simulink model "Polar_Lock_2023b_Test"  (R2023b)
settings: Solver=FixedStepDiscrete  StartTime=0.0  StopTime=inf  FixedStep=0.01  RelTol=1e-3  EnableMultiTasking=on
libraries: arduinolib x7

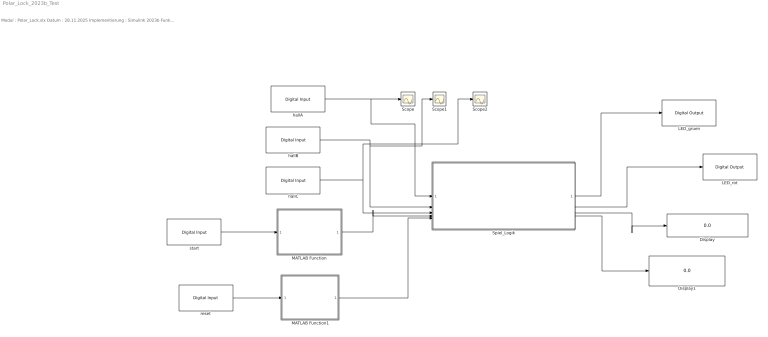
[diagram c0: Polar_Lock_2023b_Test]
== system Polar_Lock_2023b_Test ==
  note: Modul : Polar_Lock.slx Datum : 28.11.2025 Implementierung : Simulink 2023b Funktion: Autor : Yash Uppal und Barinder Singh Letzte Änderung : 28.12.2025
  Display : Display
  Display1 : Display
  LED_gruen : arduinolib/Digital Output  pinNumber=11  Direction=output  blockPlatform=arduino
  LED_rot : arduinolib/Digital Output  pinNumber=12  Direction=output  blockPlatform=arduino
  MATLAB Function : MATLAB Function  TreatAsAtomicUnit=on
  MATLAB Function1 : MATLAB Function  TreatAsAtomicUnit=on
  Scope : Scope
  Scope1 : Scope
  Scope2 : Scope
  Spiel_Logik : Subsystem
  hallA : arduinolib/Digital Input  pinNumber=3  mode=Default  Direction=input  SampleTime=0.1  blockPlatform=arduino
  hallB : arduinolib/Digital Input  pinNumber=4  mode=Default  Direction=input  SampleTime=0.1  blockPlatform=arduino
  hallC : arduinolib/Digital Input  pinNumber=6  mode=Default  Direction=input  SampleTime=0.1  blockPlatform=arduino
  reset : arduinolib/Digital Input  pinNumber=9  mode=Default  Direction=input  SampleTime=0.1  blockPlatform=arduino
  start : arduinolib/Digital Input  pinNumber=8  mode=Default  Direction=input  SampleTime=0.1  blockPlatform=arduino
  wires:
  hallA/1 -> Spiel_Logik/1(hallA), Scope/1
  hallB/1 -> Spiel_Logik/2(hallB), Scope1/1
  hallC/1 -> Spiel_Logik/3(hallC), Scope2/1
  Spiel_Logik/1(LED_gruen) -> LED_gruen/1
  Spiel_Logik/2(LED_rot) -> LED_rot/1
  Spiel_Logik/3(code) -> Display/1
  Spiel_Logik/4(status) -> Display1/1
  start/1 -> MATLAB Function/1(startRaw)
  MATLAB Function/1(startEvent) -> Spiel_Logik/4(startEvent)
  reset/1 -> MATLAB Function1/1(resetRaw)
  MATLAB Function1/1(resetDeb) -> Spiel_Logik/5(resetDeb)

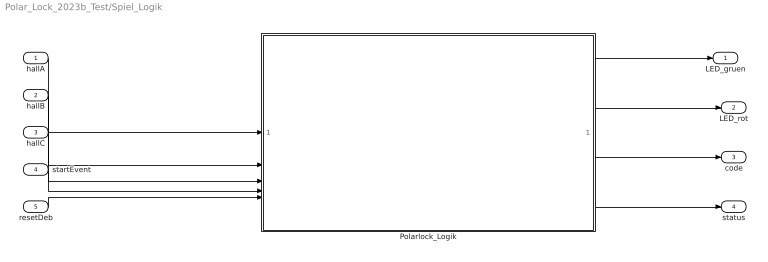
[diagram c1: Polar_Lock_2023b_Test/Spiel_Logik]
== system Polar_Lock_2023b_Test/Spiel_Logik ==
  hallA : Inport
  hallB : Inport  Port=2
  hallC : Inport  Port=3
  startEvent : Inport  Port=4
  resetDeb : Inport  Port=5
  Polarlock_Logik : MATLAB Function  TreatAsAtomicUnit=on
  LED_gruen : Outport
  LED_rot : Outport  Port=2
  code : Outport  Port=3
  status : Outport  Port=4
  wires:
  hallA/1 -> Polarlock_Logik/1(hallA)
  hallB/1 -> Polarlock_Logik/2(hallB)
  hallC/1 -> Polarlock_Logik/3(hallC)
  Polarlock_Logik/1(LED_gruen) -> LED_gruen/1
  Polarlock_Logik/2(LED_rot) -> LED_rot/1
  Polarlock_Logik/3(code) -> code/1
  Polarlock_Logik/4(status) -> status/1
  startEvent/1 -> Polarlock_Logik/4(start)
  resetDeb/1 -> Polarlock_Logik/5(reset)

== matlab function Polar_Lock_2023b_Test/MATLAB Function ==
function startEvent = DebounceStart(startRaw)
% DebounceStart
% Entprellt den Start-Taster und erzeugt einen 1-Zyklus-Impuls
% bei gültigem Tastendruck (steigende Flanke).
%
% Fixed-step size: 0.01 s
% Entprellzeit: 2 * 10 ms = 20 ms

N_DEBOUNCE = int32(2);

persistent cnt;
persistent debounced;
persistent prevDebounced;

if isempty(cnt)
    cnt = int32(0);
end
if isempty(debounced)
    debounced = int32(0);
end
if isempty(prevDebounced)
    prevDebounced = int32(0);
end

% -------- Entprellung --------
if startRaw == 1
    if cnt < N_DEBOUNCE
        cnt = cnt + 1;
    end
else
    cnt = int32(0);
    debounced = int32(0);
end

if cnt >= N_DEBOUNCE
    debounced = int32(1);
end

% -------- Flankenerkennung --------
startEvent = (debounced == 1) && (prevDebounced == 0);

prevDebounced = debounced;
end

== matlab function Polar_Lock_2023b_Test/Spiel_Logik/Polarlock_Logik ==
function [LED_gruen, LED_rot, code, status] = GameLogic(hallA, hallB, hallC, start, reset)

% Zustände
persistent state;
persistent prevA prevB prevC;
persistent stableCount;

if isempty(state)
    state = int32(0); % STATE_IDLE
end
if isempty(prevA)
    prevA = int32(-1);
    prevB = int32(-1);
    prevC = int32(-1);
end
if isempty(stableCount)
    stableCount = int32(0);
end

STATE_IDLE        = int32(0);    % LCD: "Bereit, Lege los"
STATE_CHECK       = int32(1);    % LCD: "wird geprüft"
STATE_SUCCESS     = int32(2);    % LCD: "Erfolgreich"
STATE_FAIL_LOCKED = int32(3);    % LCD: "Fehlversuch"

N_STABLE = int32(50);   % 50 Samples

% Ausgänge (Default)
LED_gruen = 0;
LED_rot   = 0;
code      = int32(0);
status    = STATE_IDLE;   % Default-LCD-Status (wird im switch passend gesetzt)

% Reset hat immer Priorität (reset ist bei dir entprellt)
if reset == 1
    state       = STATE_IDLE;
    stableCount = int32(0);
    prevA       = int32(-1);
    prevB       = int32(-1);
    prevC       = int32(-1);

    status = STATE_IDLE;  % LCD: "Bereit, Lege los"
    return;
end

switch state

    case STATE_IDLE
        LED_gruen   = 0;
        LED_rot     = 0;
        code        = int32(0);
        status      = STATE_IDLE;

        stableCount = int32(0);
        prevA       = int32(-1);
        prevB       = int32(-1);
        prevC       = int32(-1);

        if start == 1  % start ist bei dir ein Impuls (startEvent)
            state  = STATE_CHECK;
            status = STATE_CHECK;  % direkt "wird geprüft"
        end

    case STATE_CHECK
        status = STATE_CHECK;

        % Gültiges Signal = 0 (Süd) oder 1 (Nord)
        hasSignalA = (hallA == 0) || (hallA == 1);
        hasSignalB = (hallB == 0) || (hallB == 1);
        hasSignalC = (hallC == 0) || (hallC == 1);

        % Solange noch nicht alle drei ein gültiges Signal haben:
        if ~(hasSignalA && hasSignalB && hasSignalC)
            LED_gruen   = 0;
            LED_rot     = 0;
            code        = int32(0);
            stableCount = int32(0);
            prevA       = int32(hallA);
            prevB       = int32(hallB);
            prevC       = int32(hallC);
            return;
        end

        % Prüfe, ob die aktuelle Kombination unverändert ist
        if (hallA == prevA) && (hallB == prevB) && (hallC == prevC)
            stableCount = stableCount + 1;
        else
            stableCount = int32(1);
            prevA       = int32(hallA);
            prevB       = int32(hallB);
            prevC       = int32(hallC);
        end

        % Erst entscheiden, wenn die Kombination lange genug stabil war
        if stableCount < N_STABLE
            LED_gruen = 0;
            LED_rot   = 0;
            code      = int32(0);
            status    = STATE_CHECK;
            return;
        end

        % Kombination bewerten (hier: alle drei LOW = 0 ist korrekt)
        korrektA = (hallA == 0);
        korrektB = (hallB == 0);
        korrektC = (hallC == 0);

        if korrektA && korrektB && korrektC
            state     = STATE_SUCCESS;
            LED_gruen = 1;
            LED_rot   = 0;
            code      = int32(941);
            status    = STATE_SUCCESS;
        else
            state     = STATE_FAIL_LOCKED;
            LED_gruen = 0;
            LED_rot   = 1;
            code      = int32(0);
            status    = STATE_FAIL_LOCKED;
        end

    case STATE_SUCCESS
        LED_gruen = 1;
        LED_rot   = 0;
        code      = int32(941);
        status    = STATE_SUCCESS;

    case STATE_FAIL_LOCKED
        LED_gruen = 0;
        LED_rot   = 1;
        code      = int32(0);
        status    = STATE_FAIL_LOCKED;

    otherwise
        state       = STATE_IDLE;
        stableCount = int32(0);
        status      = STATE_IDLE;
end
end

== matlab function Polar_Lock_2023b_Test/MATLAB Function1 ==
function resetDeb = DebounceReset(resetRaw)
% DebounceReset
% Entprellt den Reset-Taster.
% Ausgabe ist ein stabiler Pegel (1 solange gedrückt).
%
% Fixed-step size: 0.01 s
% Entprellzeit: 2 * 10 ms = 20 ms

N_DEBOUNCE = int32(2);

persistent cnt;
persistent debounced;

if isempty(cnt)
    cnt = int32(0);
end
if isempty(debounced)
    debounced = int32(0);
end

% -------- Entprellung --------
if resetRaw == 1
    if cnt < N_DEBOUNCE
        cnt = cnt + 1;
    end
else
    cnt = int32(0);
    debounced = int32(0);
end

if cnt >= N_DEBOUNCE
    debounced = int32(1);
end

resetDeb = debounced;
end
